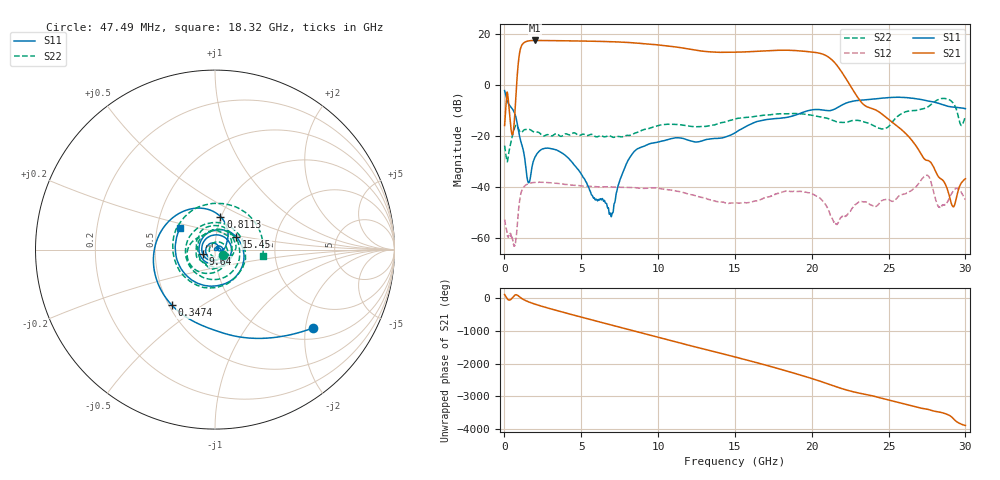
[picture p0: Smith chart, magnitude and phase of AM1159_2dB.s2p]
!Keysight Technologies,N5245B,MY58422270,A.16.20.02
!Date: Tuesday, December 10, 2024 23:09:06
!Correction: S11(C  2-Port  )
!S21(C  2-Port  )
!S12(C  2-Port  )
!S22(C  2-Port  )
!S2P File: Measurements: S11, S21, S12, S22:
# Hz S  dB  R 50
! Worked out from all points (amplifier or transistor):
!   6401 points, 10 MHz to 30 GHz, reference 50 ohm
!   highest |S21| = 17.3 dB at 1.987 GHz (marker M1)
!   |S21| within 3 dB of that: 1.054 GHz to 11.66 GHz (10.6 GHz wide, 167 % of centre)
!   unconditionally stable (mu >= 1): start of sweep to end of sweep
!   at 5.005 GHz: K = 6.61, MAG = 17.1 dB, |S12| = -39.6 dB
!   at 15.01 GHz: K = 22.16, MAG = 13.0 dB, |S12| = -46.2 dB
!   at 30 GHz: K = 5020.41, MAG = -36.0 dB, |S12| = -44.8 dB
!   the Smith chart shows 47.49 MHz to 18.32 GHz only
!   S11 on the Smith chart (normalised r, x): 47.49 MHz: 1.29, -2.20; 347.4 MHz: 0.52, -0.38; 811.3 MHz: 0.99, +0.38; 9.64 GHz: 0.87, -0.04; 15.45 GHz: 1.25, +0.18; 18.32 GHz: 0.66, +0.17
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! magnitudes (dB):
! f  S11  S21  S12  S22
! 10 MHz  -2.3  -15.9  -52.6  -23.8
! 47.49 MHz  -3.1  -12.4  -53.9  -25.6
! 347.4 MHz  -8.1  -12.3  -58.5  -24.5
! 562.9 MHz  -9.9  -18.8  -61.7  -18.8
! 811.3 MHz  -14.6  1.9  -56.8  -16.0
! 1.542 GHz  -38.1  17.1  -38.7  -17.5
! 1.987 GHz  -28.3  17.3  -38.2  -18.6
! 5.01 GHz  -35.1  17.1  -39.6  -19.5
! 6.945 GHz  -51.6  16.8  -39.9  -20.2
! 8.131 GHz  -28.7  16.5  -40.1  -19.8
! 9.64 GHz  -22.8  15.8  -40.3  -16.6
! 10.01 GHz  -22.4  15.5  -40.5  -16.0
! 15.01 GHz  -18.8  12.7  -46.2  -13.4
! 15.45 GHz  -17.2  12.8  -46.1  -13.0
! 18.32 GHz  -12.8  13.5  -41.6  -11.4
! 20 GHz  -9.9  12.8  -42.6  -11.9
! 21.58 GHz  -9.3  8.0  -54.6  -14.4
! 25 GHz  -5.0  -13.6  -44.9  -16.4
! 27.46 GHz  -6.2  -29.5  -35.4  -9.0
! 28.29 GHz  -7.4  -36.2  -47.8  -5.6
! 29.18 GHz  -8.7  -47.5  -41.8  -7.0
! 30 GHz  -9.4  -36.8  -44.8  -12.5
